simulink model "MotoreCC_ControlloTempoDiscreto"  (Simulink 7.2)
settings: Solver=ode45  StartTime=0.0  StopTime=10.0  RelTol=1e-3
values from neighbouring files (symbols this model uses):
  A = [0   1   0    [Esercitazione06.m]
  B = [0  0   1]'    [Esercitazione06.m]
  C = [1  0   0]    [Esercitazione06.m]
  Kcontr = -acker(Az,Bz,[0.9 0 0])    [Esercitazione06.m]
  Ts = 0.1    [Esercitazione06.m]
  X0 = [0.5 2 0.3]'    [Esercitazione06.m]

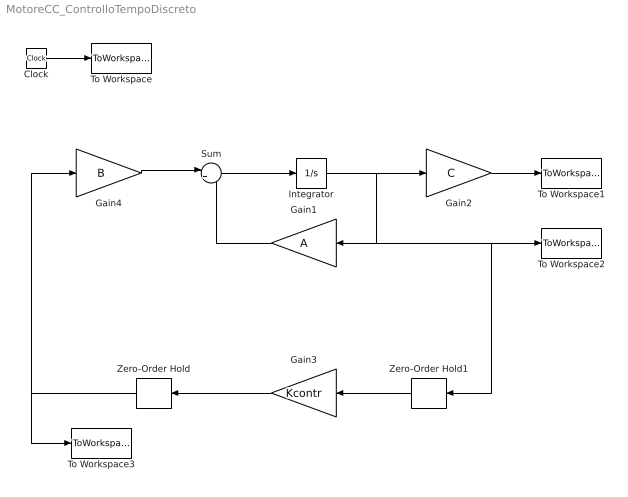
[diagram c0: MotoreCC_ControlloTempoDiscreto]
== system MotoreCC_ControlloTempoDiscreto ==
  Clock : Clock
  Gain1 : Gain  Orientation=left  Gain=A  Multiplication=Matrix(K*u)  ParameterDataType=sfix(16)  ParameterScaling=2^0  OutDataType=sfix(16)  OutScaling=2^0
  Gain2 : Gain  Gain=C  Multiplication=Matrix(K*u)  ParameterDataType=sfix(16)  ParameterScaling=2^0  OutDataType=sfix(16)  OutScaling=2^0
  Gain3 : Gain  Orientation=left  Gain=Kcontr  Multiplication=Matrix(K*u)  ParameterDataType=sfix(16)  ParameterScaling=2^0  OutDataType=sfix(16)  OutScaling=2^0  SampleTime=Ts
  Gain4 : Gain  Gain=B  Multiplication=Matrix(K*u)  ParameterDataType=sfix(16)  ParameterScaling=2^0  OutDataType=sfix(16)  OutScaling=2^0
  Integrator : Integrator  InitialCondition=X0
  Sum : Sum  Inputs=|++  OutDataType=sfix(16)  OutScaling=2^0
  To Workspace : ToWorkspace  VariableName=time  SampleTime=-1  SaveFormat=Array
  To Workspace1 : ToWorkspace  VariableName=y  SampleTime=-1  SaveFormat=Array
  To Workspace2 : ToWorkspace  VariableName=X  SampleTime=-1  SaveFormat=Array
  To Workspace3 : ToWorkspace  VariableName=ud  SampleTime=-1  SaveFormat=Array
  Zero-Order Hold : ZeroOrderHold  Orientation=left  SampleTime=Ts
  Zero-Order Hold1 : ZeroOrderHold  Orientation=left  SampleTime=Ts
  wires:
  Gain1/1 -> Sum/2
  Sum/1 -> Integrator/1
  Integrator/1 -> Gain2/1, Gain1/1, To Workspace2/1, Zero-Order Hold1/1
  Gain2/1 -> To Workspace1/1
  Gain4/1 -> Sum/1
  Gain3/1 -> Zero-Order Hold/1
  Zero-Order Hold/1 -> Gain4/1, To Workspace3/1
  Clock/1 -> To Workspace/1
  Zero-Order Hold1/1 -> Gain3/1
